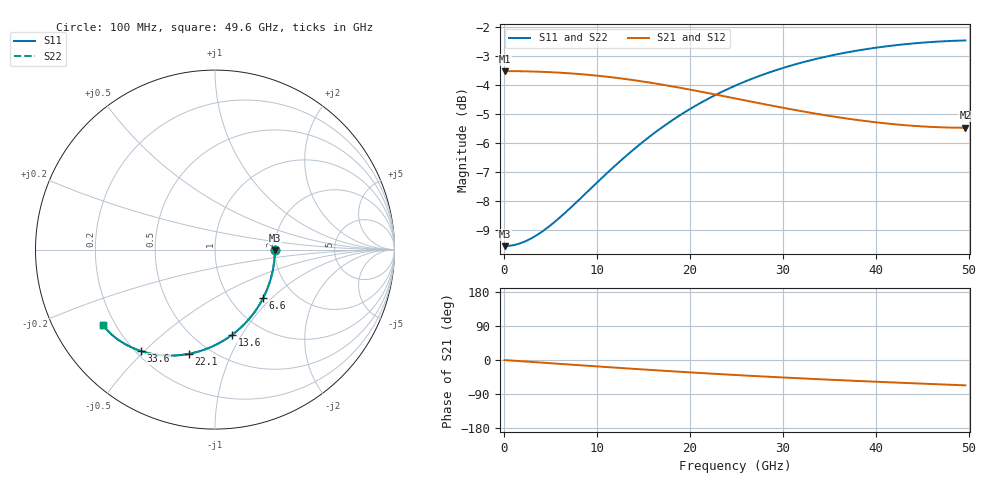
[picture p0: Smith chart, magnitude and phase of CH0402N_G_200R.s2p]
# GHz S RI R 200
! S-Parameters data
! Freq  reS11  imS11  reS21  imS21  reS12  imS12  reS22  imS22
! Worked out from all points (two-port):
!   100 points, 100 MHz to 49.6 GHz, reference 200 ohm
!   highest |S21| = -3.52 dB at 100 MHz (marker M1); lowest = -5.5 dB at 49.6 GHz (marker M2)
!   |S21| within 3 dB of the highest: start of sweep to end of sweep
!   lowest |S11| = -9.5 dB at 100 MHz (marker M3), VSWR 2.00, Z = 400 - j3.88 ohm
!   |S11| at or under -10 dB: nowhere
!   |S22| runs from -9.5 to -2.5 dB; largest |S21 - S12| = 0
!   S11 on the Smith chart (normalised r, x): 100 MHz: 2.00, -0.02; 6.6 GHz: 1.41, -0.89; 13.6 GHz: 0.74, -0.91; 22.1 GHz: 0.39, -0.70; 33.6 GHz: 0.22, -0.49; 49.6 GHz: 0.15, -0.30
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0.1  0.3333 -0.00431  0.6667 -0.00197  0.6667 -0.00197  0.3333 -0.00431
1.6  0.3293 -0.0688  0.6656 -0.0315  0.6656 -0.0315  0.3293 -0.0688
3.1  0.3184 -0.1321  0.6628 -0.0608  0.6628 -0.0608  0.3184 -0.1321
4.6  0.3009 -0.1932  0.6581 -0.0899  0.6581 -0.0899  0.3009 -0.1932
6.6  0.2684 -0.2696  0.6491 -0.128  0.6491 -0.128  0.2684 -0.2696
8.6  0.2269 -0.3387  0.637 -0.1648  0.637 -0.1648  0.2269 -0.3387
11.1  0.1655 -0.4132  0.6177 -0.2086  0.6177 -0.2086  0.1655 -0.4132
13.6  0.097 -0.4735  0.5943 -0.2491  0.5943 -0.2491  0.097 -0.4735
15.1  0.0539 -0.503  0.5787 -0.2715  0.5787 -0.2715  0.0539 -0.503
16.6  0.0103 -0.5276  0.562 -0.2924  0.562 -0.2924  0.0103 -0.5276
19.1  -0.0621 -0.5585  0.5327 -0.3239  0.5327 -0.3239  -0.0621 -0.5585
20.6  -0.1048 -0.5715  0.5144 -0.3407  0.5144 -0.3407  -0.1048 -0.5715
22.1  -0.1464 -0.5809  0.4959 -0.3561  0.4959 -0.3561  -0.1464 -0.5809
25.1  -0.2255 -0.5899  0.4587 -0.3825  0.4587 -0.3825  -0.2255 -0.5899
27.1  -0.2747 -0.5898  0.4343 -0.3974  0.4343 -0.3974  -0.2747 -0.5898
29.1  -0.3209 -0.5857  0.4103 -0.4103  0.4103 -0.4103  -0.3209 -0.5857
33.1  -0.4037 -0.5678  0.3646 -0.4314  0.3646 -0.4314  -0.4037 -0.5678
33.6  -0.4132 -0.5649  0.3591 -0.4337  0.3591 -0.4337  -0.4132 -0.5649
37.6  -0.4823 -0.5364  0.3172 -0.4499  0.3172 -0.4499  -0.4823 -0.5364
41.6  -0.54 -0.5016  0.2786 -0.4636  0.2786 -0.4636  -0.54 -0.5016
45.6  -0.5874 -0.4621  0.2427 -0.4766  0.2427 -0.4766  -0.5874 -0.4621
49.6  -0.6253 -0.4189  0.2087 -0.4902  0.2087 -0.4902  -0.6253 -0.4189
